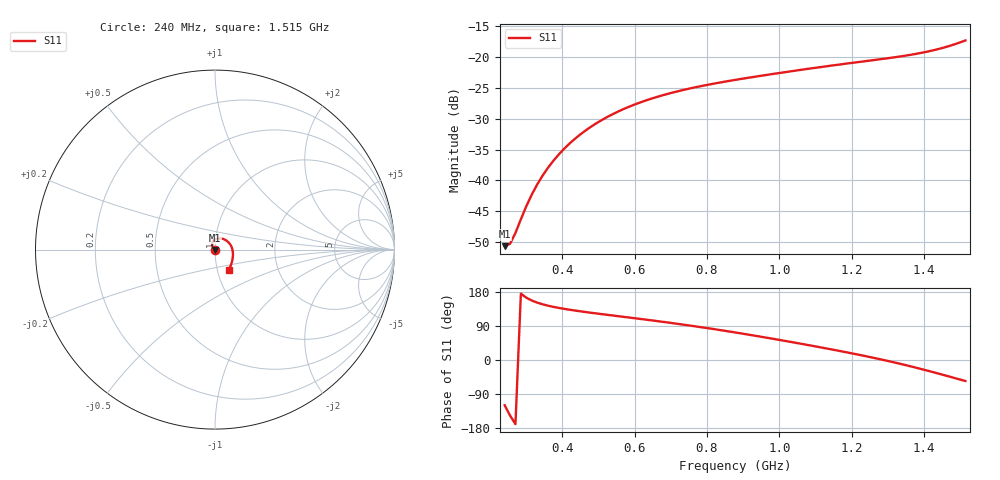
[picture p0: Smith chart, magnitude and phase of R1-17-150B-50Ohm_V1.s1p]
!version-1
!date-08.2020
!Series
#	GHZ S RI R 50.0
!	FREQ.GHZ	S11RE	S11IM
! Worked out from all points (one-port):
!   86 points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, 240 MHz to 1.515 GHz, reference 50 ohm
!   lowest |S11| = -50.6 dB at 240 MHz (marker M1), VSWR 1.01, Z = 49.9 - j0.255 ohm
!   |S11| at or under -10 dB: start of sweep to end of sweep
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0.24  -0.00143 -0.00256
0.255  -0.00256 -0.00169
0.27  -0.00369 -0.000697
0.3  -0.00595 0.00165
0.315  -0.00706 0.00299
0.33  -0.00814 0.00443
0.345  -0.00918 0.00596
0.36  -0.0102 0.00757
0.375  -0.0111 0.00926
0.405  -0.0128 0.0128
0.435  -0.0142 0.0166
0.45  -0.0147 0.0186
0.48  -0.0155 0.0226
0.525  -0.016 0.0287
0.57  -0.0153 0.0348
0.6  -0.0143 0.0388
0.645  -0.0117 0.0444
0.72  -0.00487 0.0527
0.795  0.00515 0.0589
0.885  0.0208 0.0625
1.05  0.0556 0.0548
1.125  0.0715 0.0438
1.2  0.0855 0.0273
1.29  0.0971 -0.000474
1.365  0.1 -0.0307
1.44  0.0944 -0.0679
1.485  0.0858 -0.0937
1.515  0.0775 -0.1124
